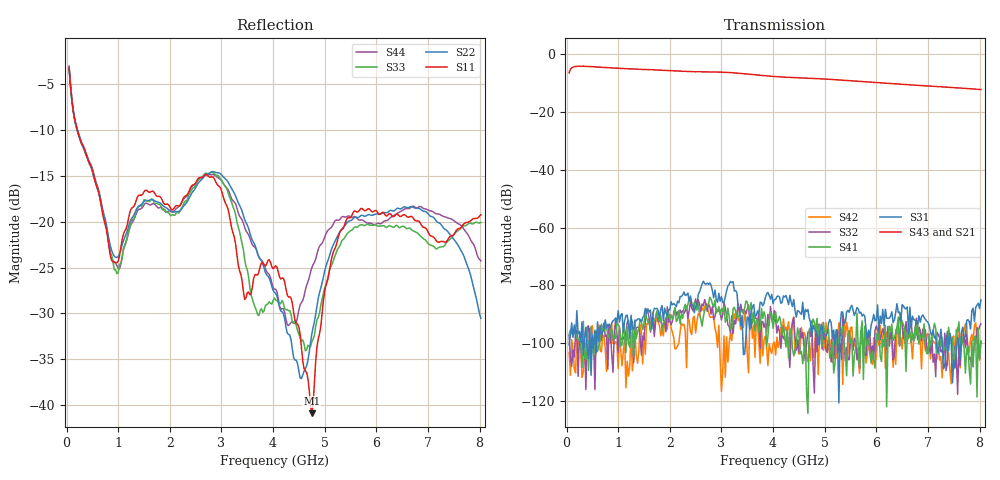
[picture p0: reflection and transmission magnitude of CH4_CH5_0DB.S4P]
!Agilent Technologies,E5071C,MY46316741,A.11.02
!Date: Mon Jun 01 11:50:16 2026
!Data & Calibration Information:
!1:CH4 INPUT 2:CH4 OUTPUT 3:CH5 INPUT 4:CH5 OUTPUT
!Freq	S11:SOLT4(ON)	S12:SOLT4(ON)	S13:SOLT4(ON)	S14:SOLT4(ON)
!	S21:SOLT4(ON)	S22:SOLT4(ON)	S23:SOLT4(ON)	S24:SOLT4(ON)
!	S31:SOLT4(ON)	S32:SOLT4(ON)	S33:SOLT4(ON)	S34:SOLT4(ON)
!	S41:SOLT4(ON)	S42:SOLT4(ON)	S43:SOLT4(ON)	S44:SOLT4(ON)
!PortZ  Port1:50+j0  Port2:50+j0  Port3:50+j0  Port4:50+j0
!Above PortZ is port z conversion or system Z0 setting when saving the data.
!When reading, reference impedance value at option line is always used.
# Hz S dB R 50
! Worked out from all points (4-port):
!   320 points, 50 MHz to 8.025 GHz, reference 50 ohm
!   strongest paths, dB at 50 MHz, 2.05 GHz, 4.05 GHz, 6.05 GHz, 8.025 GHz:
!     S43: -6.4, -5.7, -7.7, -9.8, -12.2
!     S21: -6.5, -5.8, -7.9, -10.1, -12.4
!     S31: -100.6, -86.7, -84.8, -96.7, -85.0
!     S41: -97.0, -91.6, -89.1, -94.9, -99.2
!     S32: -97.4, -92.4, -91.8, -96.0, -93.3
!     S42: -103.2, -96.2, -104.1, -100.8, -99.5
!   lowest |S11| = -40.9 dB at 4.75 GHz (marker M1), VSWR 1.02, Z = 50.3 + j0.858 ohm
!   |S11| at or under -10 dB: 208.5 MHz to end of sweep
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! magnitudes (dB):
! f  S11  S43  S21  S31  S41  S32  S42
! 50 MHz  -3.2  -6.4  -6.5  -100.6  -97.0  -97.4  -103.2
! 1 GHz  -24.3  -4.8  -5.0  -88.8  -93.7  -103.2  -108.8
! 2.85 GHz  -15.2  -6.1  -6.2  -84.3  -87.6  -91.7  -91.2
! 4.275 GHz  -28.0  -7.9  -8.2  -84.9  -95.7  -95.3  -95.6
! 4.75 GHz  -40.9  -8.3  -8.5  -97.7  -93.9  -92.3  -98.9
! 5.425 GHz  -19.7  -9.0  -9.2  -89.2  -111.3  -101.5  -92.8
! 8.025 GHz  -19.3  -12.2  -12.4  -85.0  -99.2  -93.3  -99.5
